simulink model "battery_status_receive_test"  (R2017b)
settings: Solver=FixedStepAuto  StartTime=0.0  StopTime=sim_end_time  FixedStep=fixed_step_size  RelTol=1e-3  EnableMultiTasking=on
StopFcn:
  | land1 = rospublisher('/tello1/land','std_msgs/Empty');
  | msg=rosmessage(land1);
  | send(land1,msg);
  | land2 = rospublisher('/tello2/land','std_msgs/Empty');
  | msg=rosmessage(land2);
  | send(land2,msg);
libraries: etargetslib x10, dspnetwork x10, aerolibanimutils x1

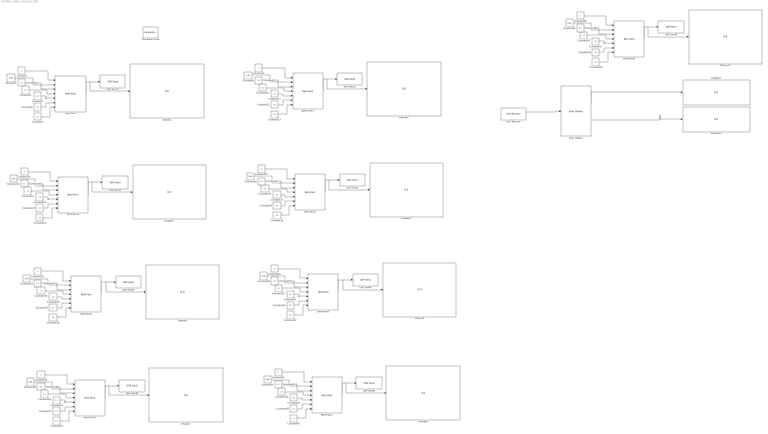
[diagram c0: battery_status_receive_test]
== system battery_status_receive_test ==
  Byte Pack{,1..8} (9 alike) : etargetslib/Byte Pack  Commented=on  datatypes={'uint8','double','double','double','double','double','double'}  byteAlign=1
  Byte Unpack : etargetslib/Byte Unpack  dimensions={[2],1}  datatypes={'uint8','double'}  byteAlign=1
  Constant : Constant  Commented=on  OutDataTypeStr=uint8
  Constant{1,8,15,26,29,40,43,54,61} (9 alike) : Constant  Commented=on  Value=0.96  OutDataTypeStr=double
  Constant{3..6,10..13,16..19,21..24,30..33,35..38,44..47,49..52,56..59} (36 alike) : Constant  Commented=on  Value=1.2  OutDataTypeStr=double
  Constant14 : Constant  Commented=on  Value=3  OutDataTypeStr=uint8
  Constant{2,9,20,27,34,41,48,55,62} (9 alike) : Constant  Commented=on  Value=0.1  OutDataTypeStr=double
  Constant25 : Constant  Commented=on  Value=4  OutDataTypeStr=uint8
  Constant28 : Constant  Commented=on  Value=5  OutDataTypeStr=uint8
  Constant39 : Constant  Commented=on  Value=6  OutDataTypeStr=uint8
  Constant42 : Constant  Commented=on  Value=7  OutDataTypeStr=uint8
  Constant53 : Constant  Commented=on  Value=8  OutDataTypeStr=uint8
  Constant60 : Constant  Commented=on  OutDataTypeStr=uint8
  Constant7 : Constant  Commented=on  Value=2  OutDataTypeStr=uint8
  Display{1..11} (11 alike) : Display
  Simulation Pace : aerolibanimutils/Simulation Pace  SimulationPace=1  SleepMode=MATLAB Thread  OutputPaceError=off  SampleTime=-1
  UDP Receive : dspnetwork/UDP Receive  localURL='0.0.0.0'  localPort=26050  remoteURL='127.0.0.1'  remotePort=-1  recvBufferSize=8192  dims=10  signalDatatype=uint8  isVarSize=off  showBlockingTime=off  blockingTime=0  sampletime=-1  blockPlatform=[]
  UDP Send1 : dspnetwork/UDP Send  Commented=on  remoteURL='127.0.0.1'  remotePort=25001  localURL='0.0.0.0'  localPortSource=Automatically determine  localPort=-1  sampletime=-1  blockPlatform=[]  separateLengthPort=0
  UDP Send2 : dspnetwork/UDP Send  Commented=on  remoteURL='127.0.0.1'  remotePort=25003  localURL='0.0.0.0'  localPortSource=Automatically determine  localPort=-1  sampletime=-1  blockPlatform=[]  separateLengthPort=0
  UDP Send3 : dspnetwork/UDP Send  Commented=on  remoteURL='127.0.0.1'  remotePort=25002  localURL='0.0.0.0'  localPortSource=Automatically determine  localPort=-1  sampletime=-1  blockPlatform=[]  separateLengthPort=0
  UDP Send4 : dspnetwork/UDP Send  Commented=on  remoteURL='127.0.0.1'  remotePort=25005  localURL='0.0.0.0'  localPortSource=Automatically determine  localPort=-1  sampletime=-1  blockPlatform=[]  separateLengthPort=0
  UDP Send5 : dspnetwork/UDP Send  Commented=on  remoteURL='127.0.0.1'  remotePort=25004  localURL='0.0.0.0'  localPortSource=Automatically determine  localPort=-1  sampletime=-1  blockPlatform=[]  separateLengthPort=0
  UDP Send6 : dspnetwork/UDP Send  Commented=on  remoteURL='127.0.0.1'  remotePort=25007  localURL='0.0.0.0'  localPortSource=Automatically determine  localPort=-1  sampletime=-1  blockPlatform=[]  separateLengthPort=0
  UDP Send7 : dspnetwork/UDP Send  Commented=on  remoteURL='127.0.0.1'  remotePort=25000  localURL='0.0.0.0'  localPortSource=Automatically determine  localPort=-1  sampletime=-1  blockPlatform=[]  separateLengthPort=0
  UDP Send8 : dspnetwork/UDP Send  Commented=on  remoteURL='127.0.0.1'  remotePort=25006  localURL='0.0.0.0'  localPortSource=Automatically determine  localPort=-1  sampletime=-1  blockPlatform=[]  separateLengthPort=0
  UDP Send9 : dspnetwork/UDP Send  Commented=on  remoteURL='127.0.0.1'  remotePort=25000  localURL='0.0.0.0'  localPortSource=Automatically determine  localPort=-1  sampletime=-1  blockPlatform=[]  separateLengthPort=0
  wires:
  Byte Pack/1 -> Display1/1, UDP Send7/1
  Constant1/1 -> Byte Pack/2
  Constant/1 -> Byte Pack/1
  Constant2/1 -> Byte Pack/3
  Constant3/1 -> Byte Pack/4
  Constant4/1 -> Byte Pack/5
  Constant5/1 -> Byte Pack/6
  Constant6/1 -> Byte Pack/7
  Constant11/1 -> Byte Pack1/5
  Constant13/1 -> Byte Pack1/7
  Constant12/1 -> Byte Pack1/6
  Constant8/1 -> Byte Pack1/2
  Constant7/1 -> Byte Pack1/1
  Constant10/1 -> Byte Pack1/4
  Constant9/1 -> Byte Pack1/3
  Byte Pack1/1 -> Display2/1, UDP Send1/1
  Constant23/1 -> Byte Pack2/6
  Constant21/1 -> Byte Pack2/4
  Constant24/1 -> Byte Pack2/7
  Constant18/1 -> Byte Pack3/6
  Constant14/1 -> Byte Pack2/1
  Constant22/1 -> Byte Pack2/5
  Constant25/1 -> Byte Pack3/1
  Constant16/1 -> Byte Pack3/4
  Constant19/1 -> Byte Pack3/7
  Byte Pack3/1 -> Display4/1, UDP Send2/1
  Constant26/1 -> Byte Pack3/2
  Constant17/1 -> Byte Pack3/5
  Constant15/1 -> Byte Pack2/2
  Constant20/1 -> Byte Pack2/3
  Byte Pack2/1 -> Display3/1, UDP Send3/1
  Constant27/1 -> Byte Pack3/3
  Constant37/1 -> Byte Pack4/6
  Constant35/1 -> Byte Pack4/4
  Constant38/1 -> Byte Pack4/7
  Constant32/1 -> Byte Pack5/6
  Constant28/1 -> Byte Pack4/1
  Constant36/1 -> Byte Pack4/5
  Constant39/1 -> Byte Pack5/1
  Constant30/1 -> Byte Pack5/4
  Constant33/1 -> Byte Pack5/7
  Byte Pack5/1 -> Display6/1, UDP Send4/1
  Constant40/1 -> Byte Pack5/2
  Constant31/1 -> Byte Pack5/5
  Constant29/1 -> Byte Pack4/2
  Constant34/1 -> Byte Pack4/3
  Byte Pack4/1 -> Display5/1, UDP Send5/1
  Constant41/1 -> Byte Pack5/3
  Constant51/1 -> Byte Pack6/6
  Constant49/1 -> Byte Pack6/4
  Constant52/1 -> Byte Pack6/7
  Constant46/1 -> Byte Pack7/6
  Constant42/1 -> Byte Pack6/1
  Constant50/1 -> Byte Pack6/5
  Constant53/1 -> Byte Pack7/1
  Constant44/1 -> Byte Pack7/4
  Constant47/1 -> Byte Pack7/7
  Byte Pack7/1 -> Display8/1, UDP Send6/1
  Constant54/1 -> Byte Pack7/2
  Constant45/1 -> Byte Pack7/5
  Constant43/1 -> Byte Pack6/2
  Constant48/1 -> Byte Pack6/3
  Byte Pack6/1 -> Display7/1, UDP Send8/1
  Constant55/1 -> Byte Pack7/3
  UDP Receive/1 -> Byte Unpack/1
  Byte Unpack/1 -> Display9/1
  Byte Unpack/2 -> Display10/1
  Byte Pack8/1 -> UDP Send9/1, Display11/1
  Constant62/1 -> Byte Pack8/3
  Constant56/1 -> Byte Pack8/4
  Constant60/1 -> Byte Pack8/1
  Constant61/1 -> Byte Pack8/2
  Constant58/1 -> Byte Pack8/6
  Constant59/1 -> Byte Pack8/7
  Constant57/1 -> Byte Pack8/5
